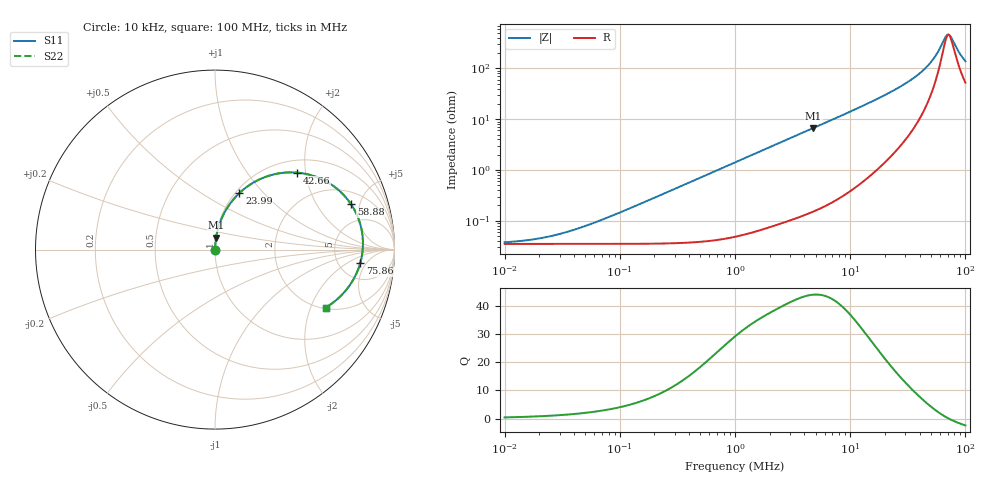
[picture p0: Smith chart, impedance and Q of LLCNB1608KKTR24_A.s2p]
! LLCNB1608KKTR24_A  S-PARAMETER MODEL  ( Standard Model )
! Model Generated by TAIYO YUDEN Corporation (http://www.ty-top.com)
! Version 1.0
! TAIYO YUDEN Control No. 170927
! Copyright(c) 2017 TAIYO YUDEN CO.,LTD. All Rights Reserved.
! Product Description (link to TY-COMPAS)
! https://ds.yuden.co.jp/TYCOMPAS/or/detail?pn=LLCNB1608KKTR24MA&u=M
! Products Name : Inductors
! Characteristics :
!  Inductance : 0.24 [uH] , SRF(min) : - [Hz] , DC Resistance(max) : 38 [mOhm]
!  Rated Current : Saturation  2.8 [A] (dL = 30 [%]), Temp Rise  2.6 [A] (dT = 40 [degC])
!  Case Size : 1.6 x 0.8 / 0.063 x 0.031 [mm/inch] , Thickness : 1.0 / 0.039 [mm/inch]
!  (Conditions: Temperature = 25 [degC] , DC Bias Current = 0 [A])
! External Node Assignments :
!  1  o---GGG---o  2
! GND o---------o GND
! Frequency Range : 10kHz  -  100MHz  [ 402 STEP ]
# MHz S RI R 50
! Freq[MHz].  S11 Real  S11 Imag  S21 Real  S21 Imag  S12 Real  S12 Imag  S22 Real  S22 Imag
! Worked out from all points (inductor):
!   401 points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, 10 kHz to 100 MHz, reference 50 ohm
!   read as one part in series: L = 224 nH near 75.86 kHz
!   highest Q = 44 at 4.786 MHz (marker M1), where L = 222 nH
!   self-resonance near 71.58 MHz
!   S11 on the Smith chart (normalised r, x): 10 kHz: 1.00, +0.00; 23.99 MHz: 1.04, +0.74; 42.66 MHz: 1.27, +1.79; 58.88 MHz: 2.96, +4.14; 75.86 MHz: 8.03, -3.61; 100 MHz: 2.05, -2.57
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0.01  0.00035 0.000141  0.9997 -0.000141  0.9997 -0.000141  0.00035 0.000141
0.021878  0.00035 0.000308  0.9997 -0.000308  0.9997 -0.000308  0.00035 0.000308
0.046774  0.00035 0.000659  0.9996 -0.000659  0.9996 -0.000659  0.00035 0.000659
0.087096  0.000352 0.00123  0.9996 -0.00123  0.9996 -0.00123  0.000352 0.00123
0.218776  0.000365 0.00308  0.9996 -0.00308  0.9996 -0.00308  0.000365 0.00308
1  0.00068 0.0141  0.9993 -0.0141  0.9993 -0.0141  0.00068 0.0141
4.677351  0.00569 0.0647  0.9943 -0.0647  0.9943 -0.0647  0.00569 0.0647
4.786301  0.00592 0.0662  0.9941 -0.0662  0.9941 -0.0662  0.00592 0.0662
10.96478  0.0276 0.1502  0.9724 -0.1502  0.9724 -0.1502  0.0276 0.1502
16.2181  0.0604 0.2197  0.9396 -0.2197  0.9396 -0.2197  0.0604 0.2197
21.87762  0.1118 0.2903  0.8882 -0.2903  0.8882 -0.2903  0.1118 0.2903
23.98833  0.1357 0.3148  0.8643 -0.3148  0.8643 -0.3148  0.1357 0.3148
32.35937  0.2564 0.3951  0.7436 -0.3951  0.7436 -0.3951  0.2564 0.3951
42.65795  0.4561 0.429  0.5439 -0.429  0.5439 -0.429  0.4561 0.429
51.28614  0.6354 0.3707  0.3646 -0.3707  0.3646 -0.3707  0.6354 0.3707
58.88437  0.7585 0.252  0.2415 -0.252  0.2415 -0.252  0.7585 0.252
66.06934  0.8173 0.1086  0.1827 -0.1086  0.1827 -0.1086  0.8173 0.1086
69.1831  0.8243 0.0459  0.1757 -0.0459  0.1757 -0.0459  0.8243 0.0459
72.4436  0.8213 -0.0165  0.1787 0.0165  0.1787 0.0165  0.8213 -0.0165
75.85776  0.809 -0.0765  0.191 0.0765  0.191 0.0765  0.809 -0.0765
89.12509  0.7121 -0.2463  0.2879 0.2463  0.2879 0.2463  0.7121 -0.2463
100  0.6166 -0.3231  0.3834 0.3231  0.3834 0.3231  0.6166 -0.3231
